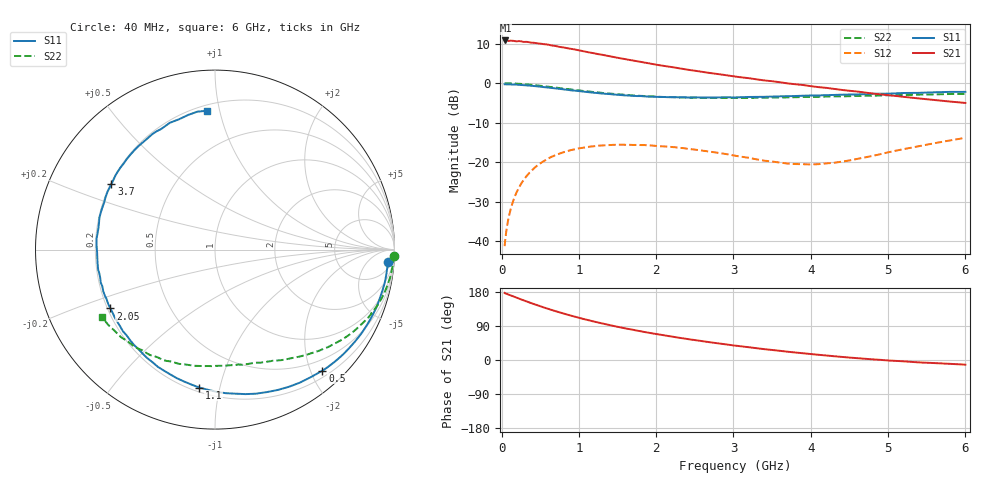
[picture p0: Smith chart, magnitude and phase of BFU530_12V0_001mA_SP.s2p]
! Filename:  P:\Prog\Test\Noise\ATS_data\Testdata_Net\03 Spar\BFU530_APG2013_40_A05_12p0V_001mA_SP_CM01_D.s2p
! Date/Time: Fri 26/Apr/2013 13:03:13
! BFU530_APG2013_40_A05_12p0V_1to25mA_SP_CM01_Bias1_R.s2p
! MDIF S-parameter v. bias file
! BFU530_APG2013_40_A05_12p0V_1to25mA_SP_CM01
! Date/time Wed Apr 24 20:41:12 2013
! bias mode 1
! bias variable = I_out
! VAR bias_var= 1
! VAR V_out= 12.0000
! VAR I_out= 0.9950
! VAR V_in= 0.7779
! VAR I_in= 0.0084
! Device data file deembeded for feedlines and parallel
! Original file: \03 Spar\BFU530_APG2013_40_A05_12p0V_001mA_SP_CM01_R.s2p
! Feed-files: PR047V01_250413_Feed1.s2p, PR047V01_250413_Feed2.s2p
! Parallel-file: PR047V01_250413_Par.s2p
# MHz S MA R 50
!  Freq-MHz  S11-mag  S11-arg  S21-mag  S21-arg  S12-mag  S12-arg  S22-mag  S22-arg
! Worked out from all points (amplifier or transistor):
!   98 points, 40 MHz to 6 GHz, reference 50 ohm
!   highest |S21| = 10.8 dB at 50 MHz (marker M1)
!   |S21| within 3 dB of that: start of sweep to 1.128 GHz
!   unconditionally stable (mu >= 1): 3.283 GHz to 4.931 GHz
!   at 300 MHz: K = 0.09, MSG = 17.3 dB, |S12| = -24.1 dB
!   at 1.6 GHz: K = 0.40, MSG = 10.8 dB, |S12| = -15.6 dB
!   at 6 GHz: K = 0.78, MSG = 4.4 dB, |S12| = -13.8 dB
!   S11 on the Smith chart (normalised r, x): 40 MHz: 11, -23; 500 MHz: 0.30, -2.19; 1.1 GHz: 0.23, -0.87; 2.05 GHz: 0.21, -0.25; 3.7 GHz: 0.20, +0.28; 6 GHz: 0.24, +0.91
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40  0.967 -4.0  3.454 177.0  0.008682 86.9  0.9969 -1.9
50  0.9659 -5.0  3.461 175.7  0.01086 86.0  0.9979 -2.5
100  0.9642 -9.9  3.411 172.0  0.0216 83.1  0.9935 -5.2
120  0.9625 -12.0  3.441 170.4  0.02585 81.9  0.9919 -6.3
200  0.9554 -19.8  3.374 164.1  0.04258 76.6  0.9834 -10.7
340  0.933 -33.5  3.309 153.4  0.06961 67.9  0.9601 -17.9
500  0.9017 -48.4  3.157 142.0  0.09652 58.5  0.9258 -25.3
600  0.8794 -57.4  3.069 135.2  0.1107 53.1  0.9015 -29.7
700  0.8564 -66.0  2.944 128.8  0.1228 47.9  0.8772 -33.8
900  0.8109 -81.9  2.711 117.0  0.1425 39.0  0.8315 -40.8
1050  0.7816 -93.0  2.54 108.8  0.1522 32.8  0.7971 -45.8
1100  0.7734 -96.5  2.48 106.2  0.1547 30.9  0.7871 -47.2
1350  0.7319 -113.0  2.232 94.3  0.1638 22.4  0.7439 -54.1
1600  0.6992 -127.9  2.01 83.5  0.1661 15.0  0.7098 -60.4
1850  0.6797 -141.1  1.818 73.8  0.1648 9.0  0.6872 -65.9
2050  0.669 -150.6  1.678 67.0  0.1593 5.1  0.6698 -70.3
2500  0.6606 -170.1  1.435 52.6  0.1445 -1.5  0.6532 -79.5
3100  0.6629 167.2  1.183 36.1  0.1174 -3.0  0.6494 -91.5
3700  0.683 147.7  0.9915 21.9  0.09611 7.0  0.6601 -103.6
4100  0.6993 136.5  0.8893 13.8  0.09448 19.8  0.6704 -111.7
5200  0.7501 109.6  0.6705 -3.5  0.1462 40.4  0.7054 -133.5
6000  0.7752 93.4  0.5614 -12.3  0.2034 38.2  0.7324 -148.9
